| TEXAS INSTRUMENTS INCORPORATED
| Standard Linear and Logic Group
| IBIS Model of SN74ALVCF162835
| 3.3-V CMOS 18-BIT UNIVERSAL BUS DRIVER WITH 3-STATE OUTPUTS
| This file contains package information for the following:
|  TSSOP 56-pin (DGG) package as [Component] ALVCF162835_DGG
|  TVSOP 56-pin (DGV) package as [Component] ALVCF162835_DGV
|  SSOP 56-pin (DL) package as [Component] ALVCF162835_DL
| This device can be powered at the following Vccs:
|  3.3 volt Vcc
|  2.5 volt Vcc
| This file provides unique models under the [Model Selector] for each Vcc.
| For operation at a specific Vcc, select the appropriate model after each
| [Model Selector] keyword.
[IBIS Ver]   3.2
[Comment char]  |_char
[File Name]   sn74alvcf162835.ibs
[File Rev]   1.1 | x_die
[Date]   July 10, 2002
[Source]   Data created from TI-SPICE simulations at TI-SLL.
[Notes]   The following is an IBIS list for the SN74ALVCF162835.
   Please contact sllibis@ti.com with questions and
   comments concerning SLL IBIS models.
   -As there is no power clamp diode in the Input, CLK, LE, and OE
   Models, we removed the Pwr Clamp table data from those
   Models.
[Disclaimer] Property of Texas Instruments Incorporated. Unauthorized
   reproduction and/or distribution is strictly prohibited.
   This product is protected under copyright law.
   Created 2002,(C) Copyright 2002, Texas Instruments
   Incorporated, All Rights Reserved
   UNLESS THERE IS A SIGNED, WRITTEN AGREEMENT TO THE
   CONTRARY, TEXAS INSTRUMENTS (TI) IS PROVIDING THE IBIS
   MODELS  AND WITHOUT ANY WARRANTY, EXPRESSED OR
   IMPLIED.  TI assumes no liability for:
   1) the accuracy of the IBIS models provided to your
   company;
   2) the proper functioning of these IBIS Models in your
   design or for any resulting applications; or
   3) infringement of patents, copyrights or intellectual
   property rights resulting from your use of these IBIS
   models.
   TI provides IBIS Models as a service to our customers.
   You and your company shall not distribute, sell or give
   these models to anyone else without prior written
   permission from TI.
   TI reserves the right to make changes to our products or
   to discontinue any semiconductor product or service
   without notice, and advises our customers to obtain the
   latest version of relevant information to verify, before
   placing orders, that the information being relied on is
   current.
   Please be aware that your receipt and use of the IBIS
   information provided shall serve as acceptance of these
   terms and conditions. If you do not accept these terms,
   you should return or destroy the IBIS models and any
   other accompanying information immediately.
| Component ALVCF162835_DGG 56-pin TSSOP
[Component]   ALVCF162835_DGG
[Manufacturer]   Texas Instruments, Inc.
[Package]
|   typ   min   max
R_pkg   5.400e-02   4.000e-02   8.300e-02
L_pkg   3.546e-09   2.838e-09   5.045e-09
C_pkg   5.580e-13   4.120e-13   7.380e-13
[Pin]   signal_name   model_name   R_pin   L_pin   C_pin
1   NC   NC   7.600e-02   5.003e-09   7.120e-13
2   NC   NC   7.600e-02   4.539e-09   7.230e-13
3   Y1   ALVCF162835_OUT   8.300e-02   4.357e-09   7.080e-13
4   GND   GND   4.200e-02   3.999e-09   6.830e-13
5   Y2   ALVCF162835_OUT   4.200e-02   3.806e-09   6.700e-13
6   Y3   ALVCF162835_OUT   4.300e-02   3.603e-09   6.160e-13
7   VCC   POWER   4.400e-02   3.440e-09   5.520e-13
8   Y4   ALVCF162835_OUT   4.600e-02   3.306e-09   5.090e-13
9   Y5   ALVCF162835_OUT   4.700e-02   3.194e-09   4.820e-13
10   Y6   ALVCF162835_OUT   4.800e-02   3.088e-09   4.630e-13
11   GND   GND   5.000e-02   2.987e-09   4.350e-13
12   Y7   ALVCF162835_OUT   5.100e-02   2.910e-09   4.230e-13
13   Y8   ALVCF162835_OUT   5.200e-02   2.894e-09   4.220e-13
14   Y9   ALVCF162835_OUT   5.300e-02   2.840e-09   4.220e-13
15   Y10   ALVCF162835_OUT   5.300e-02   2.850e-09   4.230e-13
16   Y11   ALVCF162835_OUT   5.200e-02   2.886e-09   4.210e-13
17   Y12   ALVCF162835_OUT   5.100e-02   2.883e-09   4.190e-13
18   GND   GND   5.000e-02   2.941e-09   4.300e-13
19   Y13   ALVCF162835_OUT   4.900e-02   3.031e-09   4.570e-13
20   Y14   ALVCF162835_OUT   4.700e-02   3.131e-09   4.760e-13
21   Y15   ALVCF162835_OUT   4.600e-02   3.244e-09   5.030e-13
22   VCC   POWER   4.400e-02   3.387e-09   5.500e-13
23   Y16   ALVCF162835_OUT   4.300e-02   3.566e-09   6.320e-13
24   Y17   ALVCF162835_OUT   4.200e-02   3.801e-09   6.870e-13
25   GND   GND   4.100e-02   3.961e-09   6.870e-13
26   Y18   ALVCF162835_OUT   8.100e-02   4.291e-09   7.110e-13
27   NOE   ALVCF162835_OE   7.600e-02   4.561e-09   7.380e-13
28   LE   ALVCF162835_LE   7.500e-02   5.045e-09   7.240e-13
29   GND   GND   7.300e-02   5.020e-09   7.140e-13
30   CLK   ALVCF162835_CLK   7.400e-02   4.532e-09   7.200e-13
31   A18   ALVCF162835_IN   8.300e-02   4.336e-09   7.080e-13
32   GND   GND   4.000e-02   3.957e-09   6.840e-13
33   A17   ALVCF162835_IN   4.200e-02   3.789e-09   6.800e-13
34   A16   ALVCF162835_IN   4.300e-02   3.540e-09   6.240e-13
35   VCC   POWER   4.400e-02   3.361e-09   5.460e-13
36   A15   ALVCF162835_IN   4.600e-02   3.222e-09   4.980e-13
37   A14   ALVCF162835_IN   4.700e-02   3.110e-09   4.710e-13
38   A13   ALVCF162835_IN   4.800e-02   3.012e-09   4.510e-13
39   GND   GND   5.000e-02   2.934e-09   4.230e-13
40   A12   ALVCF162835_IN   5.100e-02   2.879e-09   4.120e-13
41   A11   ALVCF162835_IN   5.200e-02   2.883e-09   4.130e-13
42   A10   ALVCF162835_IN   5.300e-02   2.847e-09   4.170e-13
43   A9   ALVCF162835_IN   5.300e-02   2.838e-09   4.170e-13
44   A8   ALVCF162835_IN   5.200e-02   2.887e-09   4.160e-13
45   A7   ALVCF162835_IN   5.100e-02   2.897e-09   4.160e-13
46   GND   GND   5.000e-02   2.965e-09   4.270e-13
47   A6   ALVCF162835_IN   4.800e-02   3.047e-09   4.550e-13
48   A5   ALVCF162835_IN   4.700e-02   3.138e-09   4.740e-13
49   A4   ALVCF162835_IN   4.600e-02   3.250e-09   5.030e-13
50   VCC   POWER   4.400e-02   3.390e-09   5.500e-13
51   A3   ALVCF162835_IN   4.300e-02   3.546e-09   6.260e-13
52   A2   ALVCF162835_IN   4.200e-02   3.783e-09   6.860e-13
53   GND   GND   4.000e-02   3.955e-09   6.820e-13
54   A1   ALVCF162835_IN   8.300e-02   4.330e-09   7.010e-13
55   NC   NC   7.700e-02   4.562e-09   7.240e-13
56   GND   GND   7.500e-02   5.029e-09   7.120e-13
| Component ALVCF162835_DGV 56-pin TVSOP
[Component]   ALVCF162835_DGV
[Manufacturer]  Texas Instruments, Inc.
[Package]
|   typ   min   max
R_pkg   6.300e-02   5.000e-02   8.600e-02
L_pkg   2.945e-09   2.392e-09   3.938e-09
C_pkg   3.910e-13   2.710e-13   5.880e-13
[Pin]   signal_name   model_name   R_pin   L_pin   C_pin
1   NC   NC   6.800e-02   3.933e-09   5.880e-13
2   NC   NC   6.800e-02   3.569e-09   5.860e-13
3   Y1   ALVCF162835_OUT   7.600e-02   3.464e-09   5.150e-13
4   GND   GND   8.600e-02   3.451e-09   4.580e-13
5   Y2   ALVCF162835_OUT   8.200e-02   3.278e-09   4.260e-13
6   Y3   ALVCF162835_OUT   7.700e-02   3.143e-09   3.870e-13
7   VCC   POWER   6.900e-02   2.971e-09   4.010e-13
8   Y4   ALVCF162835_OUT   5.000e-02   2.787e-09   3.790e-13
9   Y5   ALVCF162835_OUT   5.100e-02   2.686e-09   3.200e-13
10   Y6   ALVCF162835_OUT   5.200e-02   2.607e-09   3.160e-13
11   GND   GND   5.300e-02   2.497e-09   2.970e-13
12   Y7   ALVCF162835_OUT   5.400e-02   2.438e-09   2.920e-13
13   Y8   ALVCF162835_OUT   5.500e-02   2.412e-09   2.860e-13
14   Y9   ALVCF162835_OUT   5.500e-02   2.400e-09   2.730e-13
15   Y10   ALVCF162835_OUT   5.500e-02   2.402e-09   2.730e-13
16   Y11   ALVCF162835_OUT   5.400e-02   2.398e-09   2.840e-13
17   Y12   ALVCF162835_OUT   5.400e-02   2.407e-09   2.890e-13
18   GND   GND   5.300e-02   2.448e-09   2.930e-13
19   Y13   ALVCF162835_OUT   5.200e-02   2.548e-09   3.110e-13
20   Y14   ALVCF162835_OUT   5.100e-02   2.623e-09   3.160e-13
21   Y15   ALVCF162835_OUT   5.000e-02   2.725e-09   3.700e-13
22   VCC   POWER   6.500e-02   2.903e-09   3.940e-13
23   Y16   ALVCF162835_OUT   7.300e-02   3.086e-09   3.870e-13
24   Y17   ALVCF162835_OUT   8.200e-02   3.272e-09   4.280e-13
25   GND   GND   8.200e-02   3.394e-09   4.570e-13
26   Y18   ALVCF162835_OUT   7.100e-02   3.374e-09   5.080e-13
27   NOE   ALVCF162835_OE   6.900e-02   3.572e-09   5.810e-13
28   LE   ALVCF162835_LE   6.900e-02   3.937e-09   5.740e-13
29   GND   GND   6.900e-02   3.923e-09   5.690e-13
30   CLK   ALVCF162835_CLK   6.800e-02   3.546e-09   5.740e-13
31   A18   ALVCF162835_IN   7.400e-02   3.422e-09   5.180e-13
32   GND   GND   8.100e-02   3.395e-09   4.680e-13
33   A17   ALVCF162835_IN   8.000e-02   3.255e-09   4.310e-13
34   A16   ALVCF162835_IN   7.100e-02   3.063e-09   3.860e-13
35   VCC   POWER   6.100e-02   2.878e-09   3.900e-13
36   A15   ALVCF162835_IN   5.000e-02   2.709e-09   3.640e-13
37   A14   ALVCF162835_IN   5.100e-02   2.607e-09   3.110e-13
38   A13   ALVCF162835_IN   5.100e-02   2.532e-09   3.060e-13
39   GND   GND   5.300e-02   2.440e-09   2.890e-13
40   A12   ALVCF162835_IN   5.300e-02   2.399e-09   2.860e-13
41   A11   ALVCF162835_IN   5.400e-02   2.392e-09   2.820e-13
42   A10   ALVCF162835_IN   5.500e-02   2.399e-09   2.710e-13
43   A9   ALVCF162835_IN   5.500e-02   2.395e-09   2.710e-13
44   A8   ALVCF162835_IN   5.500e-02   2.403e-09   2.830e-13
45   A7   ALVCF162835_IN   5.400e-02   2.421e-09   2.880e-13
46   GND   GND   5.300e-02   2.472e-09   2.920e-13
47   A6   ALVCF162835_IN   5.100e-02   2.569e-09   3.090e-13
48   A5   ALVCF162835_IN   5.100e-02   2.636e-09   3.130e-13
49   A4   ALVCF162835_IN   5.000e-02   2.739e-09   3.660e-13
50   VCC   POWER   6.500e-02   2.922e-09   3.900e-13
51   A3   ALVCF162835_IN   7.200e-02   3.076e-09   3.840e-13
52   A2   ALVCF162835_IN   8.100e-02   3.249e-09   4.300e-13
53   GND   GND   8.300e-02   3.400e-09   4.550e-13
54   A1   ALVCF162835_IN   7.300e-02   3.421e-09   5.060e-13
55   NC   NC   6.900e-02   3.579e-09   5.780e-13
56   GND   GND   6.900e-02   3.938e-09   5.810e-13
| Component ALVCF162835_DL 56-pin SSOP
[Component]   ALVCF162835_DL
[Manufacturer]  Texas Instruments, Inc.
[Package]
|   typ   min   max
R_pkg   5.500e-02   4.800e-02   6.700e-02
L_pkg   6.539e-09   4.802e-09   9.746e-09
C_pkg   1.880e-13   7.600e-14   5.170e-13
[Pin]   signal_name   model_name   R_pin   L_pin   C_pin
1   NC   NC   6.400e-02   9.646e-09   5.130e-13
2   NC   NC   5.900e-02   8.723e-09   2.700e-13
3   Y1   ALVCF162835_OUT   5.900e-02   8.139e-09   2.230e-13
4   GND   GND   5.600e-02   7.554e-09   2.010e-13
5   Y2   ALVCF162835_OUT   5.400e-02   6.991e-09   1.950e-13
6   Y3   ALVCF162835_OUT   5.300e-02   6.659e-09   2.020e-13
7   VCC   POWER   5.500e-02   6.321e-09   2.070e-13
8   Y4   ALVCF162835_OUT   5.500e-02   5.942e-09   1.330e-13
9   Y5   ALVCF162835_OUT   5.700e-02   5.767e-09   1.320e-13
10   Y6   ALVCF162835_OUT   5.400e-02   5.459e-09   1.210e-13
11   GND   GND   5.100e-02   5.224e-09   1.400e-13
12   Y7   ALVCF162835_OUT   4.800e-02   5.088e-09   1.260e-13
13   Y8   ALVCF162835_OUT   5.000e-02   5.021e-09   9.600e-14
14   Y9   ALVCF162835_OUT   5.100e-02   4.802e-09   7.600e-14
15   Y10   ALVCF162835_OUT   5.100e-02   4.803e-09   7.600e-14
16   Y11   ALVCF162835_OUT   5.000e-02   5.021e-09   9.600e-14
17   Y12   ALVCF162835_OUT   4.800e-02   5.088e-09   1.260e-13
18   GND   GND   5.100e-02   5.224e-09   1.400e-13
19   Y13   ALVCF162835_OUT   5.400e-02   5.459e-09   1.210e-13
20   Y14   ALVCF162835_OUT   5.700e-02   5.768e-09   1.330e-13
21   Y15   ALVCF162835_OUT   5.500e-02   5.942e-09   1.330e-13
22   VCC   POWER   5.500e-02   6.320e-09   2.060e-13
23   Y16   ALVCF162835_OUT   5.300e-02   6.659e-09   2.030e-13
24   Y17   ALVCF162835_OUT   5.400e-02   6.991e-09   1.960e-13
25   GND   GND   5.600e-02   7.554e-09   2.010e-13
26   Y18   ALVCF162835_OUT   5.900e-02   8.139e-09   2.230e-13
27   NOE   ALVCF162835_OE   5.900e-02   8.727e-09   2.700e-13
28   LE   ALVCF162835_LE   6.700e-02   9.746e-09   5.170e-13
29   GND   GND   6.300e-02   9.630e-09   5.110e-13
30   CLK   ALVCF162835_CLK   6.000e-02   8.751e-09   2.710e-13
31   A18   ALVCF162835_IN   6.000e-02   8.184e-09   2.250e-13
32   GND   GND   5.600e-02   7.543e-09   2.000e-13
33   A17   ALVCF162835_IN   5.400e-02   7.005e-09   1.960e-13
34   A16   ALVCF162835_IN   5.600e-02   6.714e-09   2.040e-13
35   VCC   POWER   5.800e-02   6.384e-09   2.080e-13
36   A15   ALVCF162835_IN   5.700e-02   5.976e-09   1.340e-13
37   A14   ALVCF162835_IN   5.700e-02   5.743e-09   1.300e-13
38   A13   ALVCF162835_IN   5.400e-02   5.468e-09   1.190e-13
39   GND   GND   5.500e-02   5.328e-09   1.420e-13
40   A12   ALVCF162835_IN   5.200e-02   5.189e-09   1.290e-13
41   A11   ALVCF162835_IN   5.200e-02   5.053e-09   9.600e-14
42   A10   ALVCF162835_IN   5.100e-02   4.825e-09   7.600e-14
43   A9   ALVCF162835_IN   5.400e-02   4.896e-09   7.800e-14
44   A8   ALVCF162835_IN   5.200e-02   5.093e-09   9.700e-14
45   A7   ALVCF162835_IN   5.100e-02   5.179e-09   1.280e-13
46   GND   GND   5.400e-02   5.314e-09   1.420e-13
47   A6   ALVCF162835_IN   5.500e-02   5.511e-09   1.210e-13
48   A5   ALVCF162835_IN   5.700e-02   5.771e-09   1.310e-13
49   A4   ALVCF162835_IN   5.600e-02   5.957e-09   1.330e-13
50   VCC   POWER   5.500e-02   6.320e-09   2.060e-13
51   A3   ALVCF162835_IN   5.200e-02   6.621e-09   2.000e-13
52   A2   ALVCF162835_IN   5.300e-02   6.973e-09   1.950e-13
53   GND   GND   5.700e-02   7.571e-09   2.020e-13
54   A1   ALVCF162835_IN   5.700e-02   8.097e-09   2.220e-13
55   NC   NC   5.900e-02   8.723e-09   2.710e-13
56   GND   GND   6.100e-02   9.560e-09   5.090e-13
| Model ALVCF162835_LE
[Model Selector]   ALVCF162835_LE
ALVCF162835_LE_33   3.3 volt Vcc
ALVCF162835_LE_25   2.5 volt Vcc
| Model ALVCF162835_CLK
[Model Selector]   ALVCF162835_CLK
ALVCF162835_CLK_33   3.3 volt Vcc
ALVCF162835_CLK_25   2.5 volt Vcc
| Model ALVCF162835_OE
[Model Selector]   ALVCF162835_OE
ALVCF162835_OE_33   3.3 volt Vcc
ALVCF162835_OE_25   2.5 volt Vcc
| Model ALVCF162835_IN
[Model Selector]   ALVCF162835_IN
ALVCF162835_IN_33   3.3 volt Vcc
ALVCF162835_IN_25   2.5 volt Vcc
| Model ALVCF162835_OUT
[Model Selector]   ALVCF162835_OUT
ALVCF162835_OUT_33   3.3 volt Vcc
ALVCF162835_OUT_25   2.5 volt Vcc
| Models and submodels in the file (10): ALVCF162835_LE_33 (Input), ALVCF162835_LE_25 (Input), ALVCF162835_CLK_33 (Input), ALVCF162835_CLK_25 (Input), ALVCF162835_OE_33 (Input), ALVCF162835_OE_25 (Input), ALVCF162835_IN_33 (Input), ALVCF162835_IN_25 (Input), ALVCF162835_OUT_33 (3-state), ALVCF162835_OUT_25 (3-state)
